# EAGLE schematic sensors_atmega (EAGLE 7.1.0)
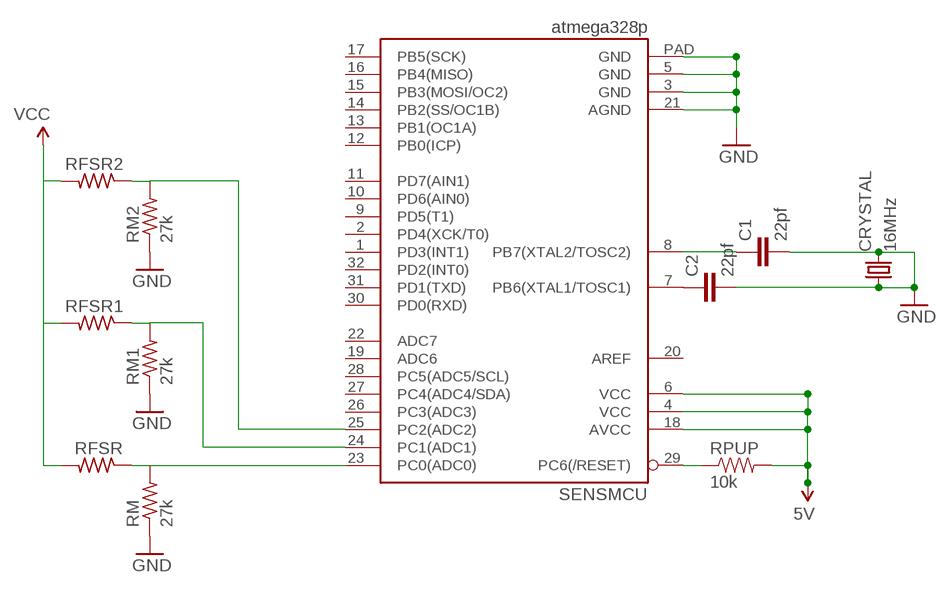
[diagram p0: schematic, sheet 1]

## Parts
C1  22pf  CAP0402-CAP  [0402-CAP]
C2  22pf  CAP0402-CAP  [0402-CAP]
CRYSTAL  16MHz  CRYSTALTC26V  [TC26V]
RFSR  R-US_M0805  [M0805]
RFSR1  R-US_M0805  [M0805]
RFSR2  R-US_M0805  [M0805]
RM  27k  R-US_M0805  [M0805]
RM1  27k  R-US_M0805  [M0805]
RM2  27k  R-US_M0805  [M0805]
RPUP  10k  RESISTOR0402-RES  [0402-RES]
SENSMCU  atmega328p  ATMEGA328P_MLFMLF32  [MLF32-PAD]

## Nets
GND: C1.2 C2.2 CRYSTAL.1 CRYSTAL.2 RM1.1 RM2.1 RM.1 SENSMCU.3(GND) SENSMCU.5(GND) SENSMCU.21(AGND) SENSMCU.PAD(GND)
N$1: RFSR.1 RM.2 SENSMCU.23(PC0(ADC0))
N$2: RFSR1.1 RM1.2 SENSMCU.24(PC1(ADC1))
N$4: RPUP.1 SENSMCU.29(PC6(/RESET))
N$5: RFSR2.1 RM2.2 SENSMCU.25(PC2(ADC2))
N$10: C1.1 SENSMCU.8(PB7(XTAL2/TOSC2))
N$11: C2.1 SENSMCU.7(PB6(XTAL1/TOSC1))
VCC: RFSR1.2 RFSR2.2 RFSR.2 RPUP.2 SENSMCU.4(VCC) SENSMCU.6(VCC) SENSMCU.18(AVCC) ; supply symbol labelled 5V
Unconnected: SENSMCU.1(PD3(INT1)) SENSMCU.2(PD4(XCK/T0)) SENSMCU.9(PD5(T1)) SENSMCU.10(PD6(AIN0)) SENSMCU.11(PD7(AIN1)) SENSMCU.12(PB0(ICP)) SENSMCU.13(PB1(OC1A)) SENSMCU.14(PB2(SS/OC1B)) SENSMCU.15(PB3(MOSI/OC2)) SENSMCU.16(PB4(MISO)) SENSMCU.17(PB5(SCK)) SENSMCU.19(ADC6) SENSMCU.20(AREF) SENSMCU.22(ADC7) SENSMCU.26(PC3(ADC3)) SENSMCU.27(PC4(ADC4/SDA)) SENSMCU.28(PC5(ADC5/SCL)) SENSMCU.30(PD0(RXD)) SENSMCU.31(PD1(TXD)) SENSMCU.32(PD2(INT0))

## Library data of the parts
C1 C2 = SparkFun-Passives:CAP: Capacitor
CRYSTAL = crystal:CRYSTAL: CRYSTAL; OC_FARNELL: unknown; OC_NEWARK: unknown
RFSR RFSR1 RFSR2 RM RM1 RM2 = resistor:R-US_: RESISTOR, American symbol
RPUP = SparkFun-Passives:RESISTOR: Resistor
SENSMCU = SparkFun-DigitalIC:ATMEGA328P_MLF: 32-Pin Atmega328 part Commonly used on Arduino compatible boards Available in QFP and QFN packages TQFP is IC-09069 QFN is non-stock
